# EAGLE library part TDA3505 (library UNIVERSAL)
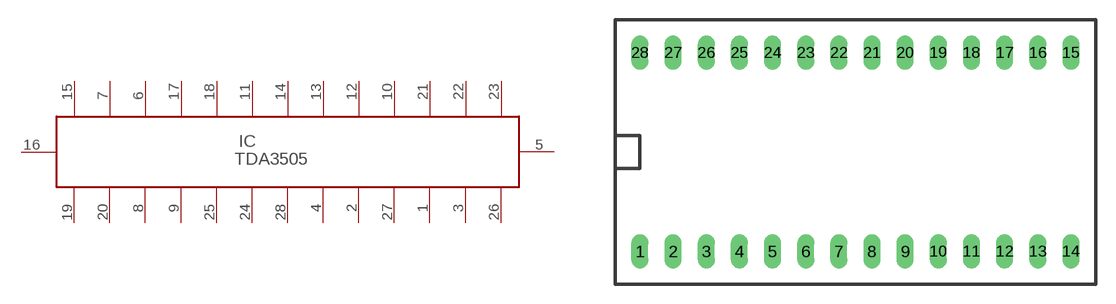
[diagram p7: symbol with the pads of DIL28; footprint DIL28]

Designator prefix IC

## TDA3505  [DIL28]
1  1
2  2
3  3
4  4
5  5
6  6
7  7
8  8
9  9
10  10
11  11
12  12
13  13
14  14
15  15
16  16
17  17
18  18
19  19
20  20
21  21
22  22
23  23
24  24
25  25
26  26
27  27
28  28

## Footprint DIL28 (pad centres in mm)
drill 0.813 pad 1.27 long: 1 0,0; 2 2.54,0; 3 5.08,0; 4 7.62,0; 5 10.16,0; 6 12.7,0; 7 15.24,0; 8 17.78,0; 9 20.32,0; 10 22.86,0; 11 25.4,0; 12 27.94,0; 13 30.48,0; 14 33.02,0; 15 33.02,15.24; 16 30.48,15.24; 17 27.94,15.24; 18 25.4,15.24; 19 22.86,15.24; 20 20.32,15.24; 21 17.78,15.24; 22 15.24,15.24; 23 12.7,15.24; 24 10.16,15.24; 25 7.62,15.24; 26 5.08,15.24; 27 2.54,15.24; 28 0,15.24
